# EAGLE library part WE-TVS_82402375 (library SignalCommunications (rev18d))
TVS Diode Standard Series Characteristics Operating temperature: –55 ºC to +85 °C for 824 023 x; –55 ºC to +125 °C for 824 021/824 022 Very low clamping voltage High ESD withstand voltage Unidirectional or bidirectional protection RoHS, REACH and free of halogens Applications DC power supply Headsets and accessories PDAs Digital cameras MP3-Player Touch Panels ESD protection in accordance with EN 61000-4-2 – 8 kV contact discharge – 15 kV air discharge Updated by Dan Xu 2014-07-11 2014 (C) Wurth Elektronik
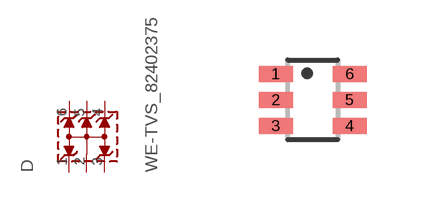
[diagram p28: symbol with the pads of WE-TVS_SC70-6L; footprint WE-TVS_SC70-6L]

Designator prefix D

## WE-TVS_82402375  [WE-TVS_SC70-6L]
1  1  pas
2  GND  pas
3  2  pas
4  3  pas
5  4  pas
6  5  pas

## Footprint WE-TVS_SC70-6L (pad centres in mm)
TVS Diode Array WE-TVS
smd 0.85 x 0.4: 1 -0.925,0.65; 2 -0.925,0; 3 -0.925,-0.65; 4 0.925,-0.65; 5 0.925,0; 6 0.925,0.65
